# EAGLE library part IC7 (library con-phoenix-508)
PHOENIX
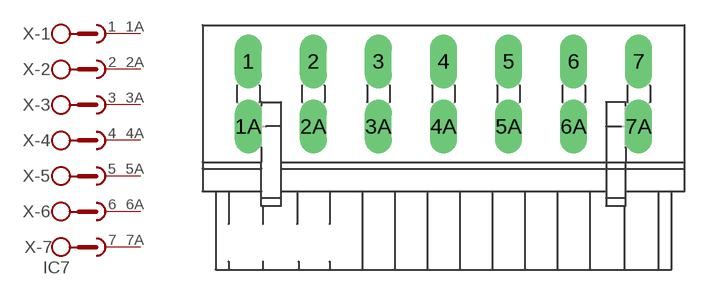
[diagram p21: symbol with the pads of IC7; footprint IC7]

Designator prefix X; gates -1=SKB2 -2=SKB2 -3=SKB2 -4=SKB2 -5=SKB2 -6=SKB2 -7=SKB2V

## IC7 (OC_FARNELL: unknown; OC_NEWARK: unknown)  [IC7]
1  -1:1  pas
1A  -1:2  pas
2  -2:1  pas
2A  -2:2  pas
3  -3:1  pas
3A  -3:2  pas
4  -4:1  pas
4A  -4:2  pas
5  -5:1  pas
5A  -5:2  pas
6  -6:1  pas
6A  -6:2  pas
7  -7:1  pas
7A  -7:2  pas

## Footprint IC7 (pad centres in mm)
PHOENIX
drill 1.397 long: 1 -15.24,2.54; 1A -15.24,-2.54; 2 -10.16,2.54; 2A -10.16,-2.54; 3 -5.08,2.54; 3A -5.08,-2.54; 4 0,2.54; 4A 0,-2.54; 5 5.08,2.54; 5A 5.08,-2.54; 6 10.16,2.54; 6A 10.16,-2.54; 7 15.24,2.54; 7A 15.24,-2.54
